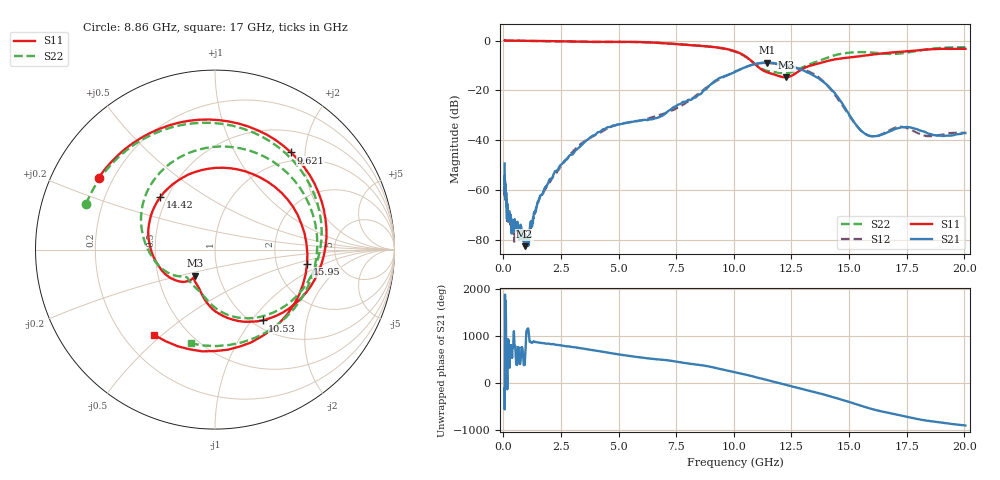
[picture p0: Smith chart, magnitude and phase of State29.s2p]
# Hz S DB R 50
!freq MagS11 AngS11 MagS21 AngS21 MagS12 AngS12 MagS22 AngS22
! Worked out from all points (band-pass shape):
!   1601 points, 50 MHz to 20.05 GHz, reference 50 ohm
!   highest |S21| = -8.83 dB at 11.43 GHz (marker M1); lowest = -82.4 dB at 918.6 MHz (marker M2)
!   |S21| within 3 dB of the highest: 10.23 GHz to 12.97 GHz (2.743 GHz wide, 23.6 % of centre)
!   lowest |S11| = -14.7 dB at 12.27 GHz (marker M3), VSWR 1.45, Z = 38.4 - j11.6 ohm
!   |S11| at or under -10 dB: 10.98 GHz to 13.35 GHz (2.365 GHz wide, 19.4 % of centre)
!   |S22| runs from -13.1 to 0.0 dB; largest |S21 - S12| = 0.019
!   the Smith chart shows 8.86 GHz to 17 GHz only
!   S11 on the Smith chart (normalised r, x): 8.86 GHz: 0.15, +0.28; 9.621 GHz: 0.84, +1.73; 10.53 GHz: 1.11, -1.14; 14.42 GHz: 0.46, +0.33; 15.95 GHz: 3.00, -0.65; 17 GHz: 0.33, -0.47
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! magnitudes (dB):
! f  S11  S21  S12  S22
! 50 MHz  0.0  -49.3  -54.9  0.0
! 53.69 MHz  0.0  -55.2  -61.6  0.0
! 57.22 MHz  0.0  -56.3  -56.9  0.0
! 135.9 MHz  0.0  -65.6  -65.1  0.0
! 148.2 MHz  0.0  -71.3  -68.3  0.0
! 163.3 MHz  0.0  -67.5  -73.0  0.0
! 369.6 MHz  0.0  -74.5  -73.6  0.0
! 471.5 MHz  0.0  -74.4  -79.4  -0.1
! 519.8 MHz  -0.1  -73.4  -72.6  -0.1
! 918.6 MHz  -0.1  -82.4  -79.0  -0.1
! 1.005 GHz  -0.1  -79.8  -80.1  -0.1
! 2.722 GHz  -0.3  -47.8  -47.7  -0.4
! 7.402 GHz  -1.3  -26.6  -27.6  -1.3
! 8.86 GHz  -2.4  -18.9  -18.5  -2.4
! 9.621 GHz  -3.3  -14.2  -14.3  -3.4
! 10.53 GHz  -6.5  -10.6  -10.6  -6.6
! 11.43 GHz  -12.7  -8.8  -9.0  -12.1
! 12.27 GHz  -14.7  -10.0  -10.1  -13.1
! 14.42 GHz  -7.5  -21.5  -22.1  -5.8
! 15.95 GHz  -5.7  -38.3  -38.4  -4.8
! 17 GHz  -4.7  -35.5  -34.9  -5.4
! 20.05 GHz  -3.3  -37.1  -37.0  -2.6
